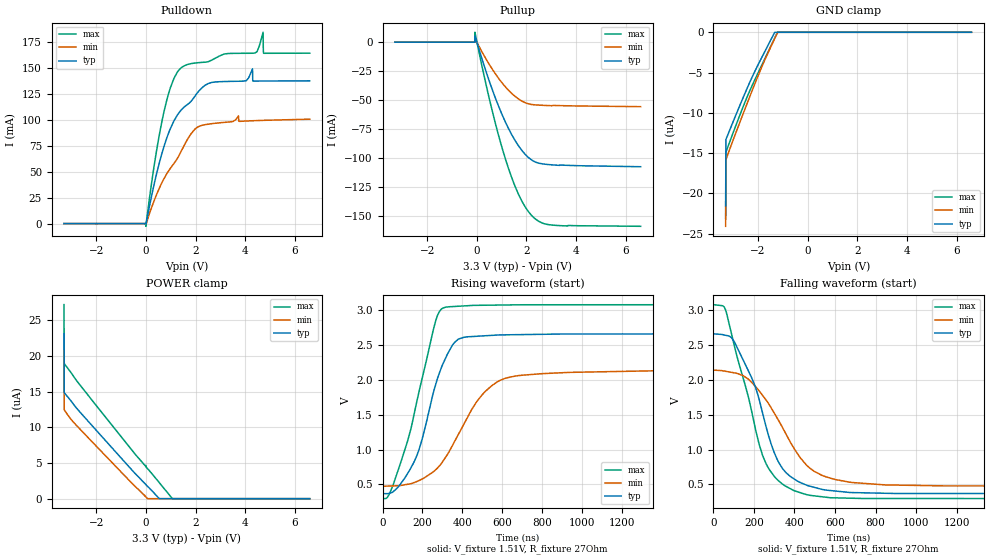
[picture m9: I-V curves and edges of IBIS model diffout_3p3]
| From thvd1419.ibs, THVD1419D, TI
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|   diffout_3p3 Model
[Model]   diffout_3p3
Model_type   I/O
Polarity   Non-Inverting
Enable   Active-High
Vinl = 0.8
Vinh = 2
Vmeas = 1.5105
Vref = 1.5105
Cref = 50pF
Rref = 27
|   typ   min   max
C_comp   801.023pF   801.023pF   801.023pF
| Where Nom  PVT is Nominal Process, 3.3V, 25C
|   Fast PVT is Strong Process,  3.6V, -40C
|   Slow PVT is Weak Process,   3.0V, 150C
[Voltage Range]   3.3   3   3.6
|Junction Temperature
[Temperature Range]   25   150   -40
[Pullup Reference]   3.3   3   3.6
[Pulldown Reference]   0   -0   0
[Power Clamp Reference]   3.3   3   3.6
[GND Clamp Reference]   0   0   0
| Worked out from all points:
|   slope of the pulldown table from 0 to 0.495 V, typ, clamps not added: 9.09 ohm
|   slope of the pullup table from 0 to 0.495 V, typ, clamps not added: 14.8 ohm
|   falling waveform, V_fixture 1.51V, R_fixture 27Ohm: 20-80 % time 160ns typ, 216ns min, 151ns max; typ from 2.65 V to 0.368 V
|   rising waveform, V_fixture 1.51V, R_fixture 27Ohm: 20-80 % time 140ns typ, 209ns min, 144ns max; typ from 0.368 V to 2.65 V
[Pulldown]
|   Voltage   I(typ)   I(min)   I(max)
-3.3V     -7.88uA    -6.87uA    -8.778uA
-3.3mV    -4.105uA   -4.239uA   -2.643mA
729.3mV   74.58mA    43.43mA    108.2mA
1.452V    110.4mA    71.32mA    151mA
2.234V    130.6mA    94.7mA     155.6mA
4.036V    137.9mA    99.01mA    164.4mA
4.293V    149.5mA    99.28mA    164.5mA
4.303V    138mA      99.29mA    164.5mA
4.392V    137.6mA    99.38mA    164.7mA
4.719V    137.6mA    99.67mA    184.7mA
4.739V    137.6mA    99.68mA    164.4mA
6.6V      137.8mA    100.8mA    164.5mA
[GND Clamp]
|   Voltage   I(typ)   I(min)   I(max)
-3.3V     -21.56uA   -24.1uA    -23.13uA
-3.29V    -13.33uA   -15.86uA   -14.9uA
-2.993V   -11.06uA   -13.33uA   -12.43uA
-2.548V   -7.766uA   -9.732uA   -8.875uA
-2.122V   -4.835uA   -6.386uA   -5.881uA
-1.736V   -2.468uA   -3.531uA   -3.37uA
-1.33V    -33.46nA   -819nA     -739.9nA
-1.211V   0A         -46.09nA   -20.32nA
6.6V      0A         0A         0A
[Pullup]
|   Voltage   I(typ)   I(min)   I(max)
-3.3V     95.64uA    90.81uA    109.2uA
-82.5mV   76.14uA    64.33uA    85.74uA
-72.6mV   75.25uA    63.41uA    8.582mA
-62.7mV   5.569mA    62.48uA    7.459mA
-42.9mV   3.547mA    2.033mA    5.358mA
570.9mV   -37.67mA   -21.43mA   -54.63mA
1.185V    -70.3mA    -39.29mA   -102.8mA
1.769V    -92.05mA   -50.18mA   -135.1mA
2.095V    -99.75mA   -53.27mA   -146.6mA
2.373V    -103.6mA   -54.11mA   -152.8mA
3.204V    -106.1mA   -54.64mA   -158.1mA
6.6V      -107.5mA   -55.63mA   -158.9mA
[POWER Clamp]
|   Voltage   I(typ)   I(min)   I(max)
-3.3V     23.13uA    20.76uA    27.21uA
-3.29V    14.87uA    12.48uA    18.95uA
-3.102V   14.08uA    11.53uA    18.07uA
-2.409V   11.18uA    8.854uA    14.86uA
-399.3mV  3.4uA      1.607uA    6.1uA
-13.2mV   2.026uA    297.5nA    4.56uA
-3.3mV    1.994uA    265.1nA    4.667uA
6.6mV     1.962uA    232.8nA    4.417uA
66mV      1.727uA    13.54nA    4.209uA
531.3mV   25.89nA    0A         2.277uA
1.066V    0A         0A         4.596nA
6.6V      0A         0A         0A
[Ramp]
R_load = 27
|   typ   min   max
dV/dt_r   1.37144/1.40127e-07   0.996161/2.09031e-07   1.66404/1.43474e-07
dV/dt_f   1.37144/1.60335e-07   0.996177/2.14024e-07   1.66405/1.50735e-07
[Falling Waveform]
V_fixture = 1.51V
V_fixture_min = 1.304V
V_fixture_max = 1.683V
R_fixture = 27Ohm
C_fixture = 0F
|   Time   V(typ)   V(min)   V(max)
0s        2.654V     2.135V     3.071V
60.59ns   2.633V     2.118V     2.992V
104.5ns   2.534V     2.095V     2.471V
185.2ns   2.05V      1.971V     1.594V
260ns     1.327V     1.708V     798.1mV
340.8ns   730.5mV    1.316V     506.1mV
457.4ns   493.7mV    784.4mV    356.7mV
597ns     407.9mV    573.8mV    309.4mV
847.1ns   374.7mV    494.1mV    299.2mV
4us       368.3mV    474.9mV    297.2mV
[Rising Waveform]
V_fixture = 1.51V
V_fixture_min = 1.304V
V_fixture_max = 1.683V
R_fixture = 27Ohm
C_fixture = 0F
|   Time   V(typ)   V(min)   V(max)
0s        368.3mV    474.9mV    297.2mV
55.23ns   402.1mV    479.9mV    511.3mV
125ns     654.6mV    502.7mV    1.116V
163.4ns   856.2mV    533mV      1.576V
267.1ns   1.938V     712.9mV    2.849V
314.3ns   2.297V     882.7mV    3.033V
380.1ns   2.578V     1.217V     3.048V
497.3ns   2.623V     1.777V     3.062V
687ns     2.642V     2.058V     3.069V
4us       2.654V     2.135V     3.071V
